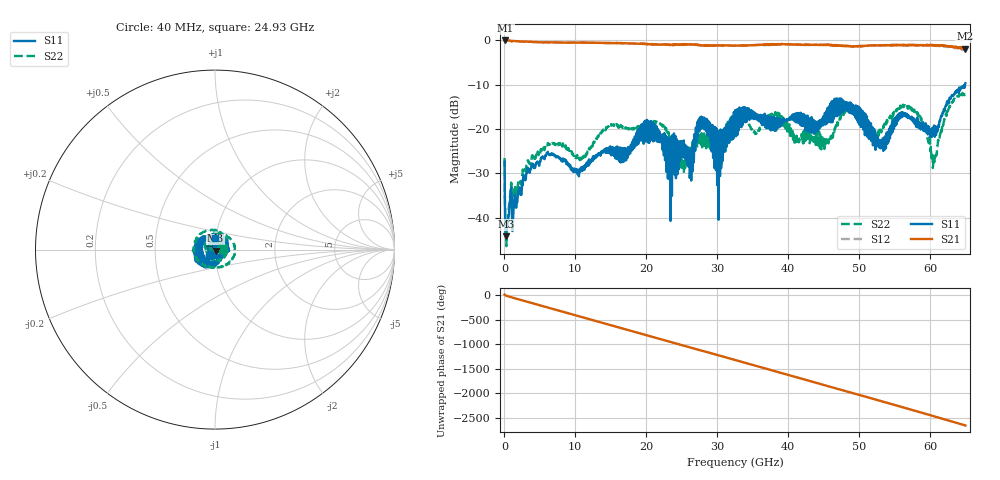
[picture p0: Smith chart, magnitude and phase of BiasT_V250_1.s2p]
! Created Tue Jul 15 19:49:34 2008
# hz S ma R 50
! 2 Port Network Data from blockName block
! freq  magS11  angS11  magS21  angS21  magS12  angS12  magS22  angS22
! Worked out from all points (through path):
!   1601 points, 40 MHz to 65 GHz, reference 50 ohm
!   highest |S21| = -0.06 dB at 161.8 MHz (marker M1); lowest = -1.9 dB at 64.92 GHz (marker M2)
!   group delay of S21, straight-line fit = 113 ps
!   lowest |S11| = -44.2 dB at 243 MHz (marker M3), VSWR 1.01, Z = 50.3 - j0.551 ohm
!   |S11| at or under -10 dB: start of sweep to 64.95 GHz
!   |S22| runs from -46.5 to -11.9 dB; largest |S21 - S12| = 0.052
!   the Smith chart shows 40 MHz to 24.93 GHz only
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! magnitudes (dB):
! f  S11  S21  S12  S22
! 40 MHz  -27.4  -0.1  -0.1  -26.6
! 161.8 MHz  -43.1  -0.1  -0.1  -41.7
! 243 MHz  -44.2  -0.1  -0.1  -42.2
! 6.089 GHz  -25.6  -0.5  -0.5  -23.6
! 10.88 GHz  -29.0  -0.5  -0.5  -26.8
! 14.86 GHz  -25.6  -0.6  -0.7  -19.3
! 21.72 GHz  -22.1  -1.0  -1.0  -18.7
! 23.34 GHz  -22.5  -1.0  -1.1  -21.3
! 25.21 GHz  -25.0  -1.0  -1.0  -27.1
! 26.23 GHz  -25.2  -1.0  -0.9  -26.4
! 27.89 GHz  -19.6  -1.2  -1.2  -24.2
! 30.33 GHz  -21.2  -1.2  -1.2  -22.6
! 32.52 GHz  -16.9  -1.2  -1.2  -17.1
! 43.36 GHz  -18.8  -1.0  -1.1  -19.8
! 45.39 GHz  -16.0  -1.1  -1.0  -22.5
! 47.79 GHz  -16.2  -1.3  -1.3  -16.5
! 54.2 GHz  -22.0  -1.1  -1.1  -17.8
! 57.94 GHz  -18.7  -1.1  -1.1  -16.3
! 60.53 GHz  -20.1  -1.1  -1.2  -27.0
! 62.69 GHz  -14.3  -1.4  -1.5  -15.4
! 64.92 GHz  -10.7  -1.9  -2.2  -12.3
! 65 GHz  -9.7  -1.8  -2.3  -12.4
